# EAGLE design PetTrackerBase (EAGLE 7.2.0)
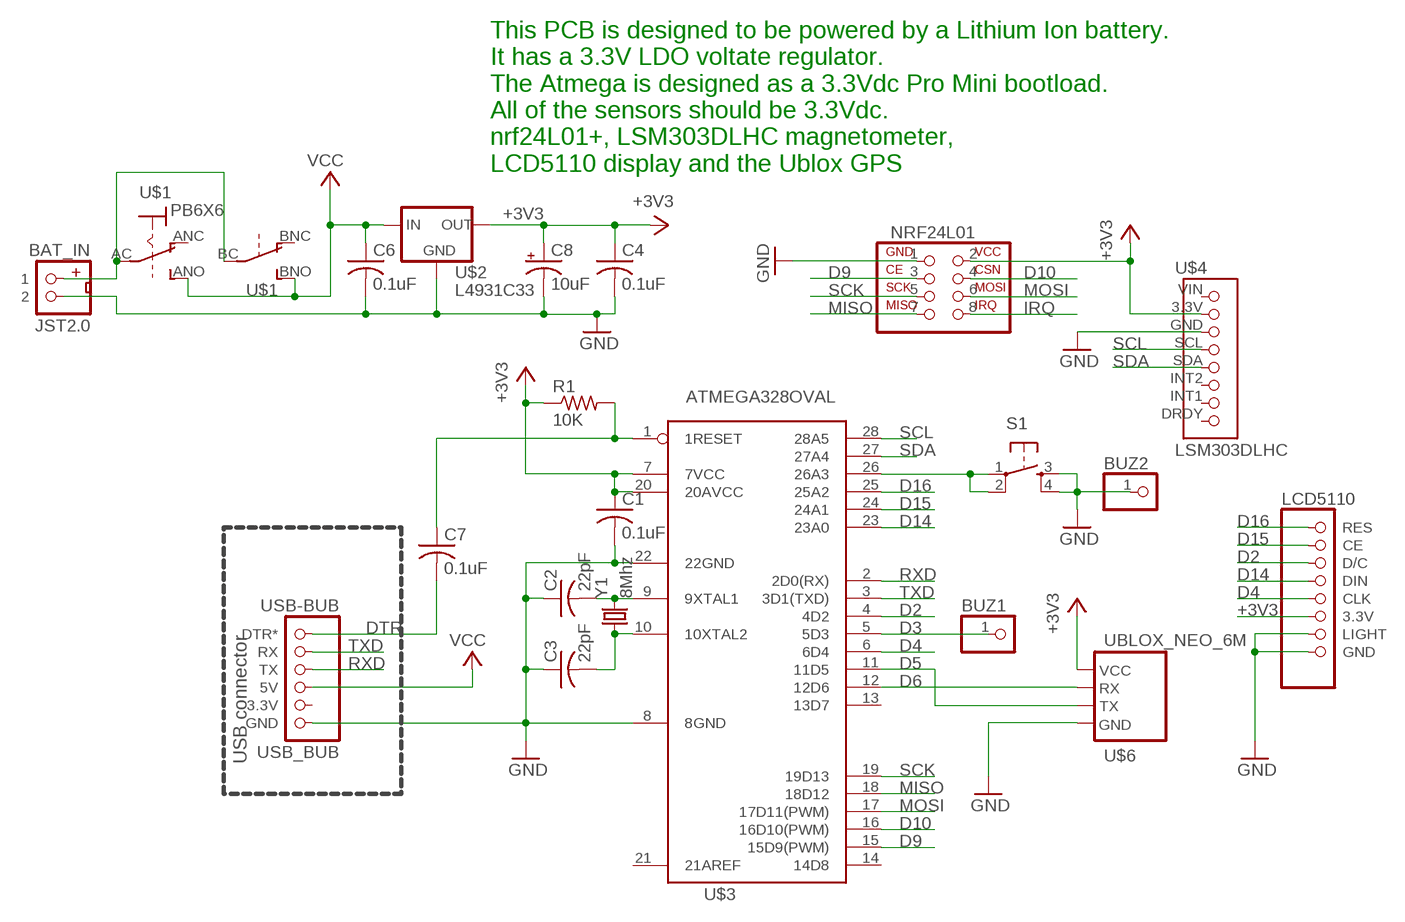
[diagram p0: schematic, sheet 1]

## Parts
BAT_IN  JST2.0  [JST2.0]
BUZ1  PINHD-1X1  [1X01]
BUZ2  PINHD-1X1  [1X01]
C1  0.1uF  C-US050-024X044  [C050-024X044]
C2  22pF  C-US025-025X050  [C025-025X050]
C3  22pF  C-US025-025X050  [C025-025X050]
C4  0.1uF  C-US025-025X050  [C025-025X050]
C6  0.1uF  C-US025-025X050  [C025-025X050]
C7  0.1uF  C-US075-042X103  [C075-042X103]
C8  10uF  CPOL-USE2.5-5V  [E2,5-4R]
LCD5110  LCD5110_1TOP  [LCD5110T1]
NRF24L01  NRF24L01+  [NRF24L01+]
R1  10K  R-US_0207/5V  [0207/5V]
S1  TAC_SWITCHPTH  [TACTILE-PTH]
U$1  PB6X6  [PB6X6]
U$2  L4931C33  [TO92-INLINE]
U$3  ATMEGA328OVAL  [DIL28-3]
U$4  LSM303DLHC  [LSM303DLHC]
U$6  UBLOX_NEO_6M  [UBLOX_NEO_6M]
USB-BUB  USB_BUB  [USB_BUB]
Y1  8Mhz  CRYSTALTC38H  [TC38H]

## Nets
+3V3: C1.1 C4.1 C8.+ LCD5110.3.3V NRF24L01.2 R1.1 U$2.1(OUT) U$3.7(7VCC) U$3.20(20AVCC) U$4.3.3V U$6.VCC
D2: LCD5110.D/C U$3.4(4D2)
D3: BUZ1.1 U$3.5(5D3)
D4: LCD5110.CLK U$3.6(6D4)
D5: U$3.11(11D5) U$6.TX
D6: U$3.12(12D6) U$6.RX
D9: NRF24L01.3 U$3.15(15D9(PWM))
D10: NRF24L01.4 U$3.16(16D10(PWM))
D14: LCD5110.DIN U$3.23(23A0)
D15: LCD5110.CE U$3.24(24A1)
D16: LCD5110.RES U$3.25(25A2)
DTR: C7.2 USB-BUB.DTR*
GND [power]: BAT_IN.2 BUZ2.1 C1.2 C2.1 C3.1 C4.2 C6.2 C8.- LCD5110.GND LCD5110.LIGHT NRF24L01.1 S1.3 S1.4 U$2.2(GND) U$3.8(8GND) U$3.22(22GND) U$4.GND U$6.GND USB-BUB.GND
IRQ: NRF24L01.8
MISO: NRF24L01.7 U$3.18(18D12)
MOSI: NRF24L01.6 U$3.17(17D11(PWM))
N$1: S1.1 S1.2 U$3.26(26A3)
N$2: BAT_IN.1 U$1.AC(P) U$1.BC(P)
N$6: C3.2 U$3.10(10XTAL2) Y1.1
N$7: C2.2 U$3.9(9XTAL1) Y1.2
RESET: C7.1 R1.2 U$3.1(1RESET)
RXD: U$3.2(2D0(RX)) USB-BUB.TX
SCK: NRF24L01.5 U$3.19(19D13)
SCL: U$3.28(28A5) U$4.SCL
SDA: U$3.27(27A4) U$4.SDA
TXD: U$3.3(3D1(TXD)) USB-BUB.RX
VCC: C6.1 U$1.ANO(S) U$1.BNO(S) U$2.3(IN) USB-BUB.5V
Unconnected: U$1.ANC(O) U$1.BNC(O) U$3.13(13D7) U$3.14(14D8) U$3.21(21AREF) U$4.DRDY U$4.INT1 U$4.INT2 U$4.VIN USB-BUB.3.3V

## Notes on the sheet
- This PCB is designed to be powered by a Lithium Ion battery. 
  It has a 3.3V LDO voltate regulator. 
  The Atmega is designed as a 3.3Vdc Pro Mini bootload.
  All of the sensors should be 3.3Vdc.
  nrf24L01+, LSM303DLHC magnetometer,
  LCD5110 display and the Ublox GPS
- USB connector

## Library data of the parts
BAT_IN = MTS_Custom:JST2.0
BUZ1 BUZ2 = pinhead:PINHD-1X1: PIN HEADER
C1-C4 C6 C7 = rcl:C-US: CAPACITOR, American symbol
C8 = rcl:CPOL-US: POLARIZED CAPACITOR, American symbol
LCD5110 = MTS_Custom:LCD5110_1
NRF24L01 = MTS_Custom:NRF24L01+
R1 = rcl:R-US_: RESISTOR, American symbol
S1 = SparkFun:TAC_SWITCH: Momentary Switch Button commonly used for reset or general input. Spark Fun Electronics SKU : COM-00097
U$1 = MTS_Custom:PB6X6: Pushbutton 6mm x 6mm DPDT. 0.5A, 50V should be the same for momentary and latching.
U$2 = MTS_Custom:L4931C33: Voltage Regulator 3.3Vdc LDO (0.4V)
U$3 = MTS_Custom:ATMEGA328
U$4 = MTS_Custom:LSM303DLHC: 3 Axis Magnetometer and 3 Axis Accelerometer Module
U$6 = MTS_Custom:UBLOX_NEO_6M
USB-BUB = MTS_Custom:USB_BUB
Y1 = crystal:CRYSTAL: CRYSTAL; OC_FARNELL: unknown; OC_NEWARK: unknown

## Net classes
0 default: width 0.305 mm
1 power: width 0.6 mm, clearance 0.3 mm

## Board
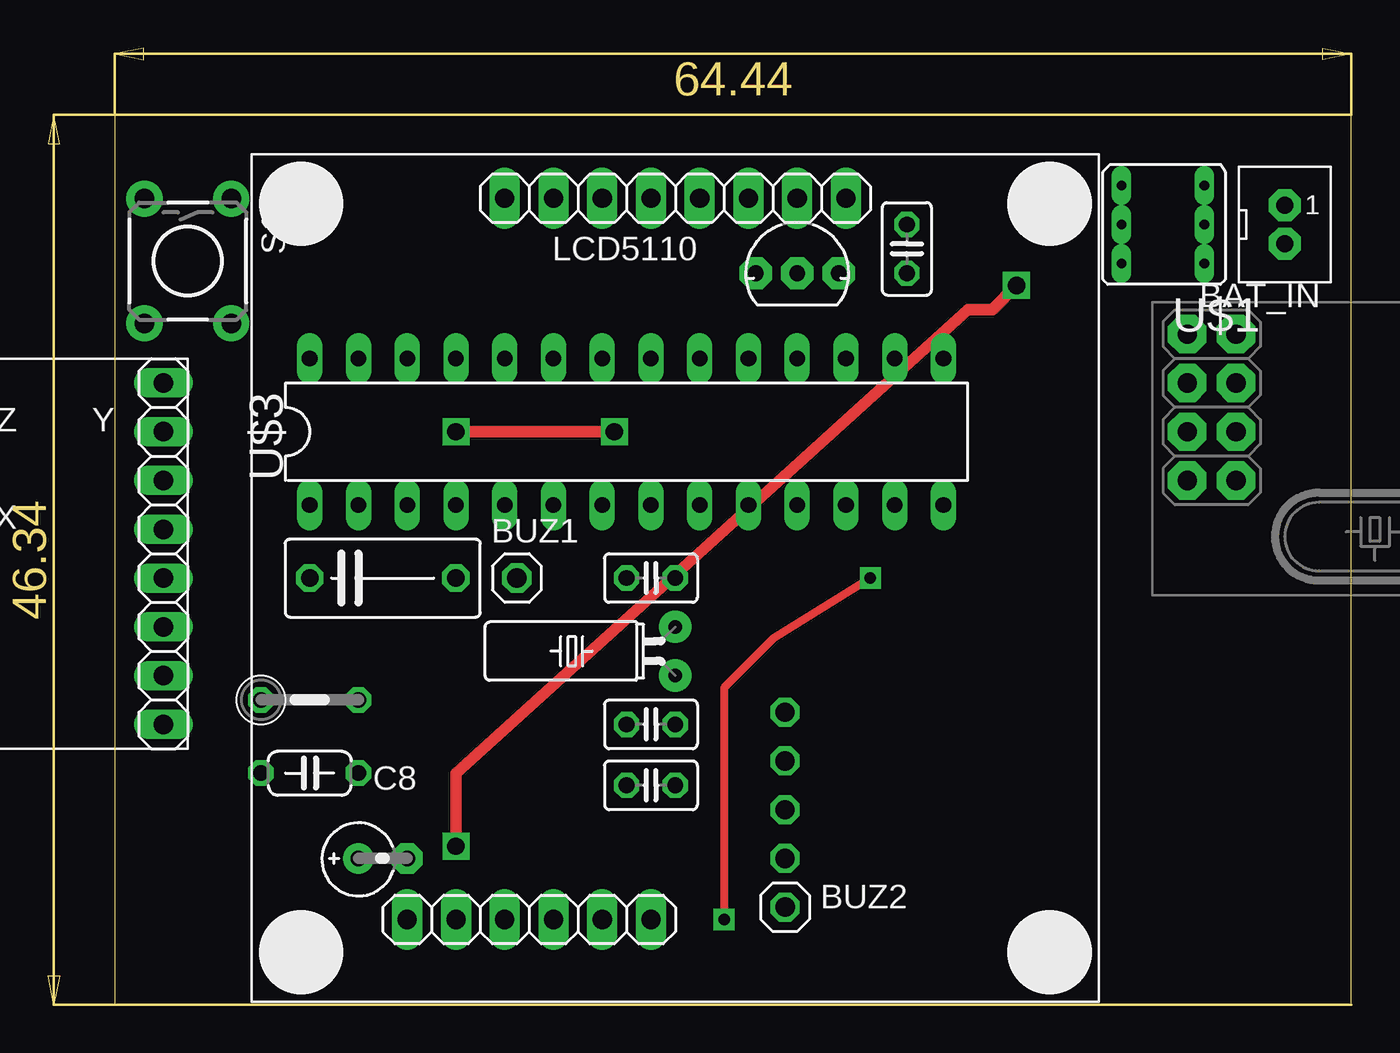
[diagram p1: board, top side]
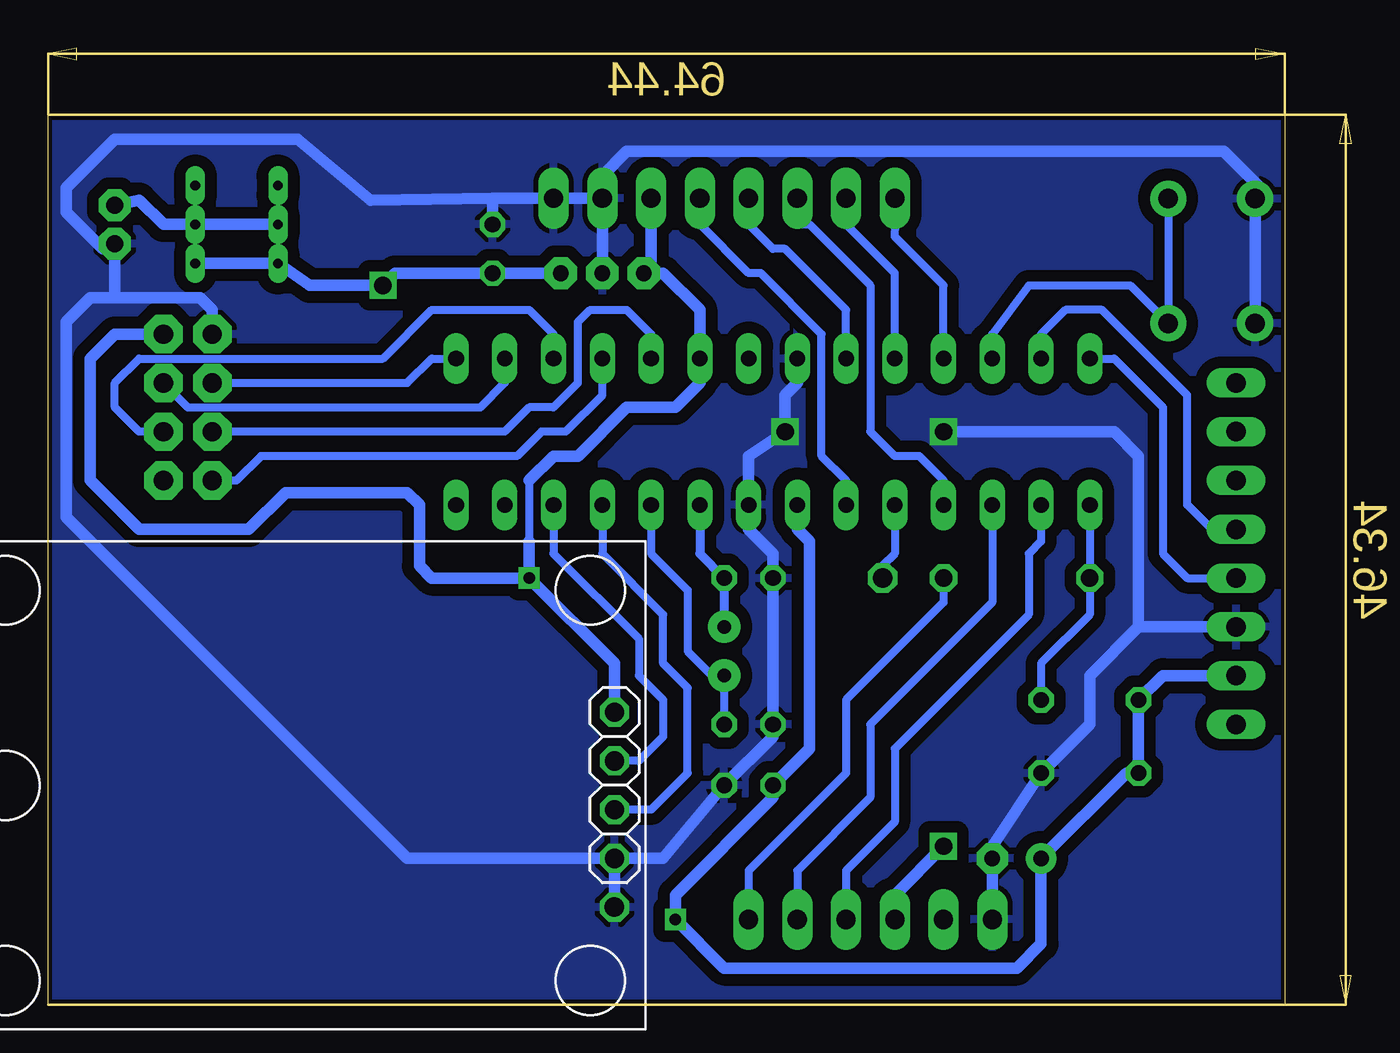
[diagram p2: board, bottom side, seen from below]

Size 67.91 x 49.83 mm. Coordinates in mm from the lower left corner, seen from the top.
Outline: 3.47,0 67.91,0 67.91,46.34 3.47,46.34 3.47,0
Copper layers (1*16): Top 0.035mm / dielectric 1.5mm / Bottom 0.035mm
Design rules "MTS": minimum track width 18mil, minimum drill 12mil, track to track 24mil, track to pad 24mil, pad to pad 6mil, via to via 6mil, smd to smd 0mil, copper to edge 8mil, drill to drill 10mil, minimum pad ring 10mil, minimum via ring 10mil, stop-mask expansion 2mil, vias tented up to drill 25mil, thermal gap 10mil

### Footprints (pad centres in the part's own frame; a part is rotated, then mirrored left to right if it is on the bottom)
JST2.0 = drill 0.9 pad 1.676 octagon: 1 0,-1; 2 0,1
1X01 = drill 1.016 octagon: 1 0,0
C050-024X044 = drill 0.813 octagon: 1 -2.54,0; 2 2.54,0
C025-025X050 = drill 0.813 octagon: 1 -1.27,0; 2 1.27,0
C075-042X103 = drill 0.914 octagon: 1 -3.81,0; 2 3.81,0
E2,5-4R = drill 0.813 pad 1.6: + -1.27,0 | drill 0.813 pad 1.6 octagon: - 1.27,0
LCD5110T1 = drill 1 pad 1.6 long: 3.3V 3.81,19.78; CE -6.35,19.78; CLK 1.27,19.78; D/C -3.81,19.78; DIN -1.27,19.78; GND 8.89,19.78; LIGHT 6.35,19.78; RES -8.89,19.78
NRF24L01+ = drill 1 pad 2 octagon: 1 -5.08,-12.7; 2 -5.08,-10.16; 3 -2.54,-12.7; 4 -2.54,-10.16; 5 0,-12.7; 6 0,-10.16; 7 2.54,-12.7; 8 2.54,-10.16
0207/5V = drill 0.813 octagon: 1 -2.54,0; 2 2.54,0
TACTILE-PTH = drill 1.016 pad 1.88: 1 -3.251,2.261; 2 3.251,2.261; 3 -3.251,-2.261; 4 3.251,-2.261
PB6X6 = drill 0.5 pad 0.813 long: AC -2.159,0; ANC -2.159,-2.032; ANO -2.159,2.032; BC 2.159,0; BNC 2.159,-2.032; BNO 2.159,2.032
TO92-INLINE = drill 0.813 pad 1.676 octagon: 1 -2.159,0; 2 0,0; 3 2.159,0
DIL28-3 = drill 0.813 long: 1 -16.51,-3.81; 2 -13.97,-3.81; 3 -11.43,-3.81; 4 -8.89,-3.81; 5 -6.35,-3.81; 6 -3.81,-3.81; 7 -1.27,-3.81; 8 1.27,-3.81; 9 3.81,-3.81; 10 6.35,-3.81; 11 8.89,-3.81; 12 11.43,-3.81; 13 13.97,-3.81; 14 16.51,-3.81; 15 16.51,3.81; 16 13.97,3.81; 17 11.43,3.81; 18 8.89,3.81; 19 6.35,3.81; 20 3.81,3.81; 21 1.27,3.81; 22 -1.27,3.81; 23 -3.81,3.81; 24 -6.35,3.81; 25 -8.89,3.81; 26 -11.43,3.81; 27 -13.97,3.81; 28 -16.51,3.81
LSM303DLHC = drill 1.016 long: 3.3V -2.54,5.08; DRDY -2.54,-10.16; GND -2.54,2.54; INT1 -2.54,-7.62; INT2 -2.54,-5.08; SCL -2.54,0; SDA -2.54,-2.54; VIN -2.54,7.62
UBLOX_NEO_6M = drill 1 octagon: GND -16.51,3.81; RX -16.51,-1.27; TX -16.51,1.27; VCC -16.51,-3.81
USB_BUB = drill 1 pad 1.6 long: 3.3V -3.81,0; 5V -1.27,0; DTR* 6.35,0; GND -6.35,0; RX 3.81,0; TX 1.27,0
TC38H = drill 0.7 pad 1.676: 1 -1.27,0; 2 1.27,0

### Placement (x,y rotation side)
BAT_IN  64.44,40.64 180 top
BUZ1  24.43,22.23 0 top
BUZ2  38.4,5.08 0 top
C1  13.63,12.06 0 top
C2  31.41,22.23 0 top
C3  31.41,14.61 0 top
C4  31.41,11.43 0 top
C6  44.75,39.37 90 top
C7  17.44,22.23 0 top
C8  17.44,7.62 0 top
LCD5110  32.68,22.23 0 top
NRF24L01  72.05,29.84 270 top
R1  13.63,15.88 0 top
S1  7.28,38.73 270 top
U$1  58.08,40.64 180 top
U$2  39.03,38.1 0 top
U$3  30.14,29.84 0 top
U$4  3.47,22.23 180 top
U$6  54.91,11.43 180 bottom
USB-BUB  25.06,4.45 0 top
Y1  32.68,18.41 90 top

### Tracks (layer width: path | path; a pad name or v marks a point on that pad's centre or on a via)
+3V3  (via drill 0.6)
  Top 0.406: v42.84,22.23 37.76,19.05 35.22,16.51 v35.22,4.45
  Bottom 0.406: 42.84,27.3 42.84,24.13
  Bottom 0.61: 42.84,27.3 41.57,28.57 40.3,28.57 37.76,31.11 35.22,31.11 33.95,32.38 U$3.20 33.95,36.2 35.86,38.1 U$2.1 36.49,38.48 LCD5110.3.3V | NRF24L01.2 64.44,34.92 65.7,33.66 65.7,27.3 63.16,24.77 57.45,24.77 55.54,26.67 49.19,26.67 48.56,26.04 48.56,22.86 47.92,22.23 v42.84,22.23 | U$4.3.3V 9.82,17.14 R1.1 C1.1 11.73,12.06 C8.+ 16.17,3.17 17.44,1.91 32.68,1.91 v35.22,4.45 35.22,5.71 30.14,10.79 C4.1 28.24,13.34 28.24,24.13 28.87,24.77 U$3.7 | v42.84,22.23 38.4,17.78 U$6.VCC | 42.84,24.13 v42.84,22.23
D2
  Bottom 0.406: LCD5110.D/C 28.87,40.64 28.24,40.64 25.06,37.47 25.06,29.84 23.79,28.57 22.52,28.57 21.25,27.3 U$3.4
D3
  Bottom 0.406: U$3.5 23.79,23.5 24.43,22.86 BUZ1.1
D4
  Bottom 0.406: U$3.6 26.33,27.3 27.6,28.57 27.6,34.92 30.78,38.1 31.41,38.1 33.95,40.64 LCD5110.CLK
D5
  Bottom 0.406: U$3.11 39.03,23.5 35.86,20.32 35.86,17.78 34.59,16.51 34.59,12.06 36.49,10.16 U$6.TX
D6
  Bottom 0.406: U$3.12 41.57,23.5 37.13,19.05 37.13,17.14 35.86,15.88 35.86,13.97 37.13,12.7 U$6.RX
D9
  Bottom 0.406: NRF24L01.3 49.19,32.38 47.92,33.66 U$3.15
D10
  Bottom 0.406: NRF24L01.4 60.62,31.11 45.38,31.11 44.11,32.38 U$3.16
D14
  Bottom 0.406: U$3.23 26.33,36.2 29.51,39.37 30.14,39.37 31.41,40.64 LCD5110.DIN
D15
  Bottom 0.406: U$3.24 23.79,38.1 26.33,40.64 LCD5110.CE
D16
  Bottom 0.406: U$3.25 21.25,37.47 23.79,40.01 23.7,41.91 LCD5110.RES
DTR
  Bottom 0.406: C7.2 21.25,20.95 26.33,15.88 26.33,12.06 31.41,6.99 USB-BUB.DTR*
GND  (via drill 0.9)
  Top 0.61: v21.25,29.84 v29.51,29.84
  Bottom 0.6: U$3.8 31.41,24.77 30.14,23.5 C2.1
  Bottom 0.61: U$3.22 28.87,32.38 29.51,31.75 v29.51,29.84 31.41,28.57 U$3.8 | LCD5110.LIGHT LCD5110.GND 44.75,42.01 | USB-BUB.GND C8.- 18.71,8.26 C1.2 13.63,14.61 13.63,17.14 11.09,19.68 | v21.25,29.84 12.36,29.84 11.09,28.57 11.09,19.68 | S1.4 S1.3 4.74,42.27 4.74,42.55 6.65,44.45 37.76,44.45 39.03,43.18 LCD5110.LIGHT | 11.09,19.68 U$4.GND | U$6.GND 49.19,7.62 66.97,25.4 66.97,35.56 65.7,36.83 64.44,36.83 | LCD5110.LIGHT U$2.2 | BUZ2.1 U$6.GND | C2.1 C3.1 30.14,13.97 C4.2 35.86,7.62 U$6.GND | C6.2 44.75,42.01 | 64.44,36.83 59.99,36.83 59.35,36.2 NRF24L01.1 | 64.44,36.83 BAT_IN.2 65.07,39.37 66.97,41.27 66.97,42.55 64.44,45.09 54.91,45.09 51.1,41.91 44.75,42.01
  pour Bottom: 2.2,-0.64 2.2,47.62 69.52,47.62 69.52,-0.64
MISO
  Bottom 0.406: NRF24L01.7 58.08,27.3 56.81,28.57 43.48,28.57 42.21,29.84 40.94,29.84 39.03,31.75 U$3.18
MOSI
  Bottom 0.406: NRF24L01.6 63.16,29.84 64.44,31.11 64.44,32.38 63.16,33.66 50.46,33.66 47.92,36.2 42.84,36.2 41.57,34.92 U$3.17
N$1
  Bottom 0.406: S1.1 S1.2 11.53,37.47 16.81,37.47 18.71,34.92 U$3.26
N$2
  Bottom 0.61: BAT_IN.1 63.16,41.91 61.89,40.64 U$1.AC U$1.BC
N$6
  Bottom 0.406: U$3.10 36.49,23.5 34.59,21.59 34.59,18.41 33.32,17.14 Y1.1 C3.2
N$7
  Bottom 0.457: U$3.9 33.95,23.5 C2.2 Y1.2
RESET
  Bottom 0.406: U$3.1 C7.1 13.63,20.32 16.17,17.78 R1.2
RXD
  Bottom 0.406: U$3.2 16.17,24.13 16.81,23.5 16.81,20.32 23.79,13.34 23.79,9.53 26.33,6.99 USB-BUB.TX
SCK
  Bottom 0.406: U$3.19 36.49,34.92 37.76,36.2 39.67,36.2 40.3,35.56 40.3,32.38 41.57,31.11 42.84,31.11 44.11,29.84 NRF24L01.5
SCL
  Bottom 0.406: U$3.28 12.36,33.66 9.82,31.11 9.82,23.5 8.55,22.23 U$4.SCL
SDA
  Bottom 0.406: U$4.SDA 7.28,24.77 8.55,26.04 8.55,31.75 13,36.2 14.9,36.2 16.17,34.92 U$3.27
TXD
  Bottom 0.406: U$3.3 18.71,20.95 25.06,14.61 25.06,10.79 28.87,6.99 USB-BUB.RX
VCC  (via drill 0.9)
  Top 0.61: v21.25,8.26 21.25,12.06 47.92,36.2 49.19,36.2 v50.46,37.47
  Bottom 0.61: USB-BUB.5V 23.79,5.71 v21.25,8.26 | U$2.3 C6.1 49.83,38.1 v50.46,37.47 54.27,37.47 U$1.BNO U$1.ANO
